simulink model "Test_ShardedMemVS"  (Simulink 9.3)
settings: Solver=VariableStepAuto  StartTime=0.0  StopTime=2  RelTol=1e-3
InitFcn:
  | Test_LibVishia_Inspc.Test_SharedMemVS_init()
libraries: libVishia_Inspc x3, libVishia_Ctrl x3, libVishia_CtrlSfn x2

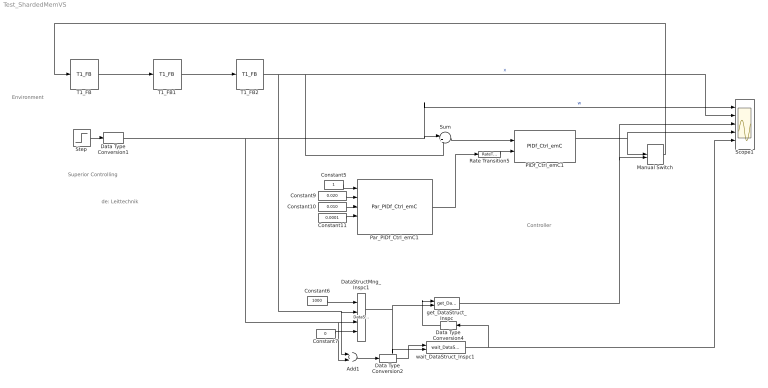
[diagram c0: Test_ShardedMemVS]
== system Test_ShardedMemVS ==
  note: Environment
  note: Controller
  note: Superior Controlling
  note: de: Leittechnik
  Add1 : Sum
  Constant10 : Constant  Value=0.010  OutDataTypeStr=single  SampleTime=-1
  Constant11 : Constant  Value=0.0001  OutDataTypeStr=single  SampleTime=-1
  Constant5 : Constant  OutDataTypeStr=single  SampleTime=-1
  Constant6 : Constant  Value=1000  OutDataTypeStr=int32  SampleTime=-1
  Constant7 : Constant  Value=0  OutDataTypeStr=single  SampleTime=-1
  Constant9 : Constant  Value=0.020  OutDataTypeStr=single  SampleTime=-1
  Data Type Conversion1 : DataTypeConversion  OutDataTypeStr=single
  Data Type Conversion2 : DataTypeConversion
  Data Type Conversion4 : DataTypeConversion
  DataStructMng_Inspc1 : libVishia_Inspc/DataStructMng_Inspc  dirGenSource='test/cpp/SharedMemExmpl/genSrc'  typeData='SPEdata'  inherit=off  chain=off  inputs=|
      | $testVishiaInspc;  //max. 15 Character
      | =step: I;     //step variable as semaphore
      | x: F;           //some input variables to C level
      | w: F;
      | =y: F;        //and one output variable from C level
  Manual Switch : ManualSwitch
  PIDf_Ctrl_emC1 : libVishia_CtrlSfn/PIDf_Ctrl_emC  Tstep=Tstep
  Par_PIDf_Ctrl_emC1 : libVishia_CtrlSfn/Par_PIDf_Ctrl_emC  Tparam=Tparam  Tctrl=Tstep  yMax=2.4  openLoop=0
  Rate Transition5 : RateTransition  OutPortSampleTimeOpt=Inherit  OutPortSampleTime=Tinit
  Scope1 : Scope  NumInputPorts=5
  Step : Step  SampleTime=0
  Sum : Sum  Inputs=|+-
  T1_FB : libVishia_Ctrl/T1_FB  T1=0.010  y0=0  Tstep=Tstep
  T1_FB1 : libVishia_Ctrl/T1_FB  T1=0.010  y0=0  Tstep=Tstep
  T1_FB2 : libVishia_Ctrl/T1_FB  T1=0.010  y0=0  Tstep=Tstep
  get_DataStruct_Inspc : libVishia_Inspc/get_DataStruct_Inspc  show='y'  Tstep=Tstep  name1='y :F'  headerfile=''
  wait_DataStruct_Inspc1 : libVishia_Inspc/wait_DataStruct_Inspc  show='step'  Tstep=Tstep  usWait=10  msTimeout=100  name1='step :I'  headerfile=''
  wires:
  T1_FB/2 -> T1_FB1/1
  T1_FB1/2 -> T1_FB2/1
  Constant9/1 -> Par_PIDf_Ctrl_emC1/2
  Rate Transition5/1 -> PIDf_Ctrl_emC1/2
  Constant11/1 -> Par_PIDf_Ctrl_emC1/4
  Data Type Conversion1/1 -> Add1/2, DataStructMng_Inspc1/3, Scope1/1, Sum/1  "w"
  Par_PIDf_Ctrl_emC1/1 -> Rate Transition5/1
  Constant5/1 -> Par_PIDf_Ctrl_emC1/1
  Constant10/1 -> Par_PIDf_Ctrl_emC1/3
  T1_FB2/2 -> Add1/1, DataStructMng_Inspc1/2, Sum/2, Scope1/2  "x"
  Sum/1 -> PIDf_Ctrl_emC1/1
  Step/1 -> Data Type Conversion1/1
  get_DataStruct_Inspc/1 -> Manual Switch/2, Scope1/3
  Constant6/1 -> DataStructMng_Inspc1/1
  Constant7/1 -> DataStructMng_Inspc1/4
  DataStructMng_Inspc1/1 -> wait_DataStruct_Inspc1/2, get_DataStruct_Inspc/2
  Add1/1 -> Data Type Conversion2/1
  Data Type Conversion2/1 -> wait_DataStruct_Inspc1/1
  wait_DataStruct_Inspc1/1 -> Data Type Conversion4/1, Scope1/5
  PIDf_Ctrl_emC1/1 -> Manual Switch/1, Scope1/4
  Manual Switch/1 -> T1_FB/1
  Data Type Conversion4/1 -> get_DataStruct_Inspc/1
